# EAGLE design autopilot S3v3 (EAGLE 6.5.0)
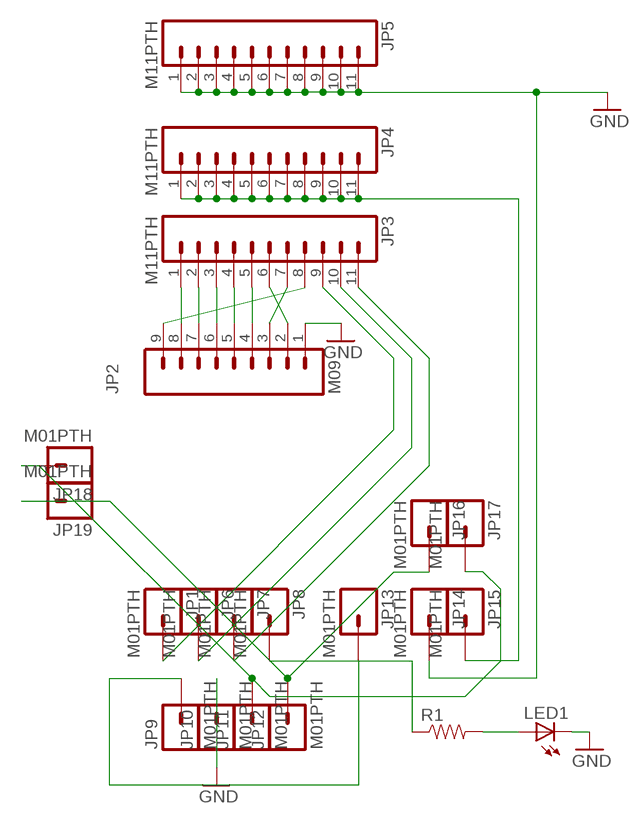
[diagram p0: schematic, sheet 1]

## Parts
JP1  M01PTH  [1X01]
JP2  M09  [1X09]
JP3  M11PTH  [1X11]
JP4  M11PTH  [1X11]
JP5  M11PTH  [1X11]
JP6  M01PTH  [1X01]
JP7  M01PTH  [1X01]
JP8  M01PTH  [1X01]
JP9  M01PTH  [1X01]
JP10  M01PTH  [1X01]
JP11  M01PTH  [1X01]
JP12  M01PTH  [1X01]
JP13  M01PTH  [1X01]
JP14  M01PTH  [1X01]
JP15  M01PTH  [1X01]
JP16  M01PTH  [1X01]
JP17  M01PTH  [1X01]
JP18  M01PTH  [1X01]
JP19  M01PTH  [1X01]
LED1  LED1206  [LED-1206]
R1  RESISTOR1206  [1206]

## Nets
GND: JP2.1 JP5.1 JP5.2 JP5.3 JP5.4 JP5.5 JP5.6 JP5.7 JP5.8 JP5.9 JP5.10 JP5.11 JP10.1 JP14.1 LED1.C
N$1: JP1.1 JP3.9
N$2: JP4.1 JP4.2 JP4.3 JP4.4 JP4.5 JP4.6 JP4.7 JP4.8 JP4.9 JP4.10 JP4.11 JP15.1
N$3: JP2.8 JP3.1
N$4: JP2.7 JP3.2
N$5: JP2.6 JP3.3
N$6: JP2.5 JP3.4
N$7: JP2.4 JP3.5
N$8: JP2.3 JP3.7
N$9: JP2.2 JP3.6
N$10: JP9.1 JP13.1
N$11: JP3.10 JP6.1
N$12: JP3.11 JP7.1
N$13: JP2.9 JP3.8
N$14: JP8.1 R1.1
N$15: LED1.A R1.2
N$16: JP11.1 JP17.1 JP18.1
N$17: JP12.1 JP16.1 JP19.1

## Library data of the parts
JP1 JP6-JP19 = SparkFun-Connectors:M01: Header 1
JP2 = SparkFun-Connectors:M09: Header 9 Standard 9-pin 0.1" header. Use with straight break away headers (SKU : PRT-00116), right angle break away headers (PRT-00553), swiss pins (PRT-00743), machine pins (PRT-00117), and female headers (PRT-00115).
JP3-JP5 = SparkFun-Connectors:M11: Header 11 Standard 11-pin 0.1" header. Use with straight break away headers (SKU : PRT-00116), right angle break away headers (PRT-00553), swiss pins (PRT-00743), machine pins (PRT-00117), and female headers (PRT-00115).
LED1 = SparkFun-LED:LED: LEDs
R1 = SparkFun-Resistors:RESISTOR: Resistor

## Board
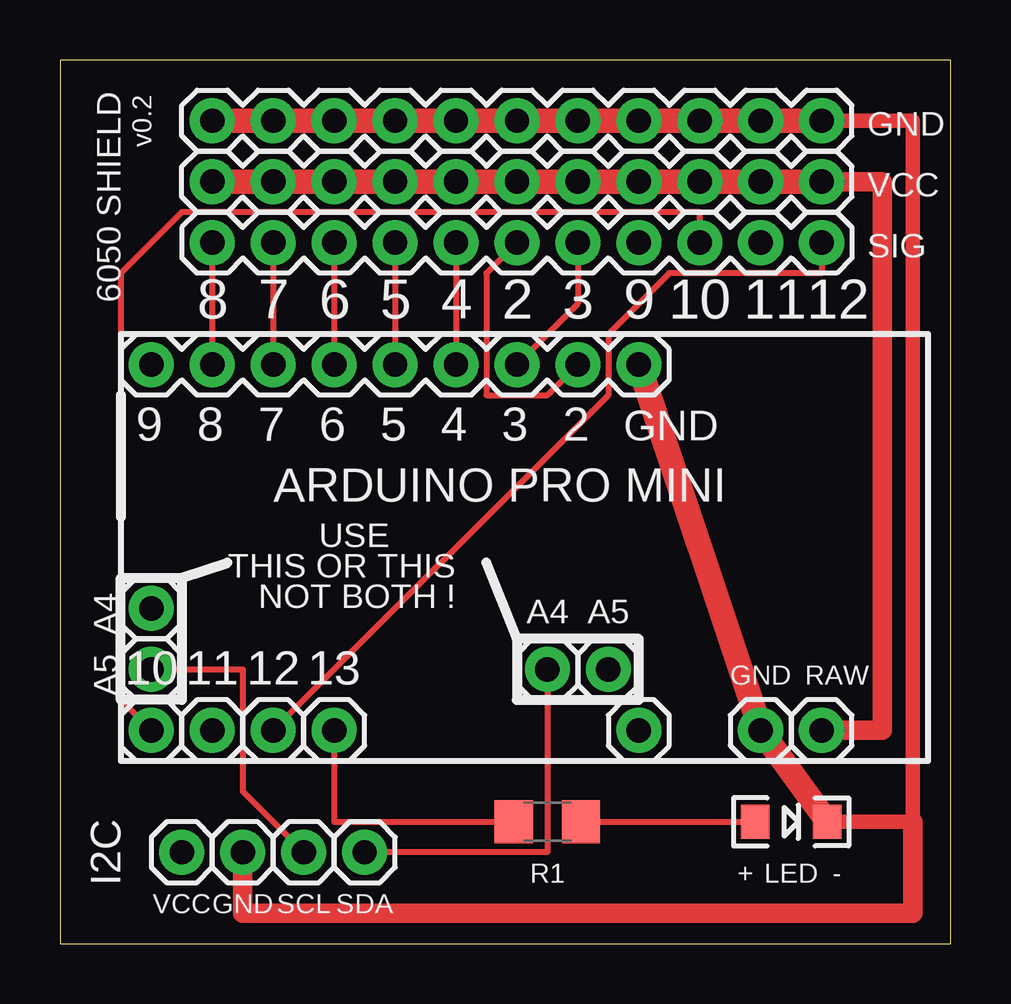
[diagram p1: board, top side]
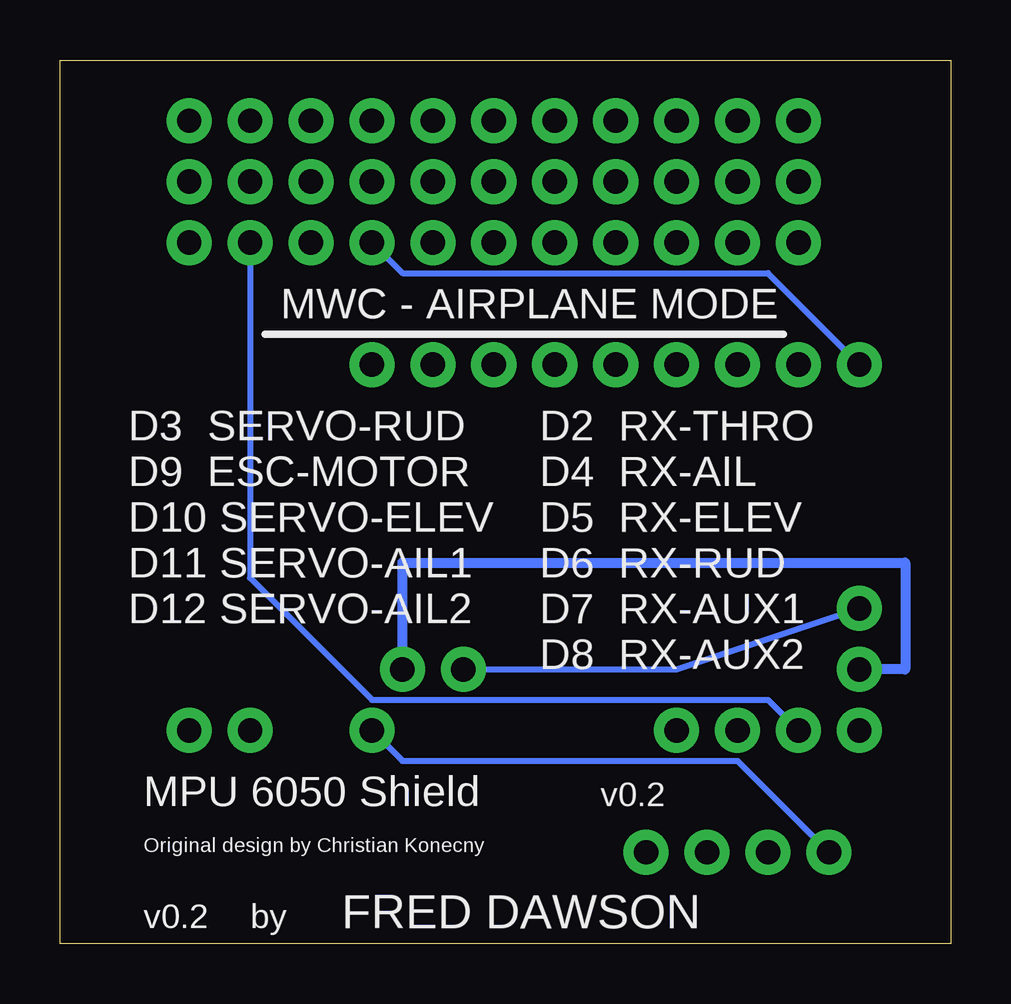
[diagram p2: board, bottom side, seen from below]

Size 37.13 x 36.82 mm. Coordinates in mm from the lower left corner, seen from the top.
Outline: 0,0 37.13,0 37.13,36.82 0,36.82 0,0
Copper layers (1*16): Top 0.035mm / dielectric 1.5mm / Bottom 0.035mm
Design rules "default": minimum track width 10mil, minimum drill 24mil, track to track 8mil, track to pad 8mil, pad to pad 8mil, via to via 8mil, smd to smd 8mil, copper to edge 40mil, drill to drill 8mil, minimum pad ring 10mil, minimum via ring 8mil, stop-mask expansion 4mil, vias tented up to drill 0mil, thermal gap 10mil

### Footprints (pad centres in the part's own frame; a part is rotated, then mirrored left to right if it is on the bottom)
1X01 = drill 1.016 pad 1.88: 1 0,0
1X09 = drill 1.016 pad 1.88: 1 0,0; 2 2.54,0; 3 5.08,0; 4 7.62,0; 5 10.16,0; 6 12.7,0; 7 15.24,0; 8 17.78,0; 9 20.32,0
1X11 = drill 1.016 pad 1.88: 1 0,0; 2 2.54,0; 3 5.08,0; 4 7.62,0; 5 10.16,0; 6 12.7,0; 7 15.24,0; 8 17.78,0; 9 20.32,0; 10 22.86,0; 11 25.4,0
LED-1206 = smd 1.2 x 1.4: A -1.5,0; C 1.5,0
1206 = smd 1.6 x 1.8: 1 -1.4,0; 2 1.4,0

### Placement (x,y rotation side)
JP1  3.81,8.89 0 top
JP2  24.13,24.13 180 top
JP3  6.35,29.21 0 top
JP4  31.75,31.75 180 top
JP5  31.75,34.29 180 top
JP6  6.35,8.89 0 top
JP7  8.89,8.89 0 top
JP8  11.43,8.89 0 top
JP9  5.08,3.81 0 top
JP10  7.62,3.81 0 top
JP11  10.16,3.81 0 top
JP12  12.7,3.81 0 top
JP13  24.13,8.89 0 top
JP14  29.21,8.89 0 top
JP15  31.75,8.89 0 top
JP16  20.32,11.43 0 top
JP17  22.86,11.43 0 top
JP18  3.81,11.43 0 top
JP19  3.81,13.97 0 top
LED1  30.48,5.08 0 top
R1  20.32,5.08 0 top

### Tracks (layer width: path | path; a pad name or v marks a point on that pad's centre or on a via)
GND
  Top 0.61: JP5.1 35.56,34.29 35.56,5.08 LED1.C
  Top 0.813: JP10.1 7.62,1.27 35.56,1.27 35.56,5.08
  Top 1.016: JP5.11 JP5.10 JP5.9 JP5.8 JP5.7 JP5.6 JP5.5 JP5.4 JP5.3 JP5.2 JP5.1 | LED1.C JP14.1 JP2.1
N$1
  Top 0.254: JP1.1 2.54,10.16 2.54,27.94 5.08,30.48 26.67,30.48 JP3.9
N$2
  Top 0.813: JP4.1 34.29,31.75 34.29,8.89 JP15.1
  Top 1.016: JP4.11 JP4.10 JP4.9 JP4.8 JP4.7 JP4.6 JP4.5 JP4.4 JP4.3 JP4.2 JP4.1
N$3
  Top 0.254: JP3.1 JP2.8
N$4
  Top 0.254: JP3.2 JP2.7
N$5
  Top 0.254: JP3.3 JP2.6
N$6
  Top 0.254: JP3.4 JP2.5
N$7
  Top 0.254: JP3.5 JP2.4
N$8
  Top 0.254: JP2.3 21.59,26.67 JP3.7
N$9
  Top 0.254: JP2.2 20.32,22.86 17.78,22.86 17.78,27.94 JP3.6
N$10
  Bottom 0.254: JP9.1 8.89,7.62 22.86,7.62 JP13.1
N$11
  Bottom 0.254: JP6.1 7.62,10.16 24.13,10.16 29.21,15.24 JP3.10
N$12
  Top 0.254: JP7.1 22.86,22.86 22.86,25.4 25.4,27.94 31.75,27.94 JP3.11
N$13
  Bottom 0.254: JP2.9 7.62,27.94 22.86,27.94 JP3.8
N$14
  Top 0.254: JP8.1 11.43,5.08 R1.1 19.05,5.08
N$15
  Top 0.254: 29.21,5.08 LED1.A R1.2 21.59,5.08
N$16
  Top 0.254: JP11.1 7.62,6.35 7.62,11.43 JP18.1
  Bottom 0.406: JP17.1 22.86,15.88 1.91,15.88 1.91,11.43 JP18.1
N$17
  Top 0.254: JP12.1 20.32,3.81 JP16.1
  Bottom 0.254: JP19.1 11.43,11.43 JP16.1

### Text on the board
tPlace: v0.2 | GND | 6050 SHIELD | VCC | SIG | 8 | 7 | 6 | 5 | 4 | 2 | 3 | 9 | 10 | 11 | 12 | 9 | 8 | 7 | 6 | 5 | 4 | 3 | 2 | GND | ARDUINO PRO MINI | USE | A4 | THIS OR THIS | NOT BOTH ! | A4 | A5 | A5 | 10 | 11 | 12 | 13 | GND | RAW | I2C | R1 | + | LED | - | VCC | GND | SCL | SDA
bPlace: MWC - AIRPLANE MODE | D2 RX-THRO | D3 SERVO-RUD | D4 RX-AIL | D9 ESC-MOTOR | D5 RX-ELEV | D10 SERVO-ELEV | D6 RX-RUD | D11 SERVO-AIL1 | D7 RX-AUX1 | D12 SERVO-AIL2 | D8 RX-AUX2 | v0.2 | MPU 6050 Shield | Original design by Christian Konecny | FRED DAWSON | by | v0.2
